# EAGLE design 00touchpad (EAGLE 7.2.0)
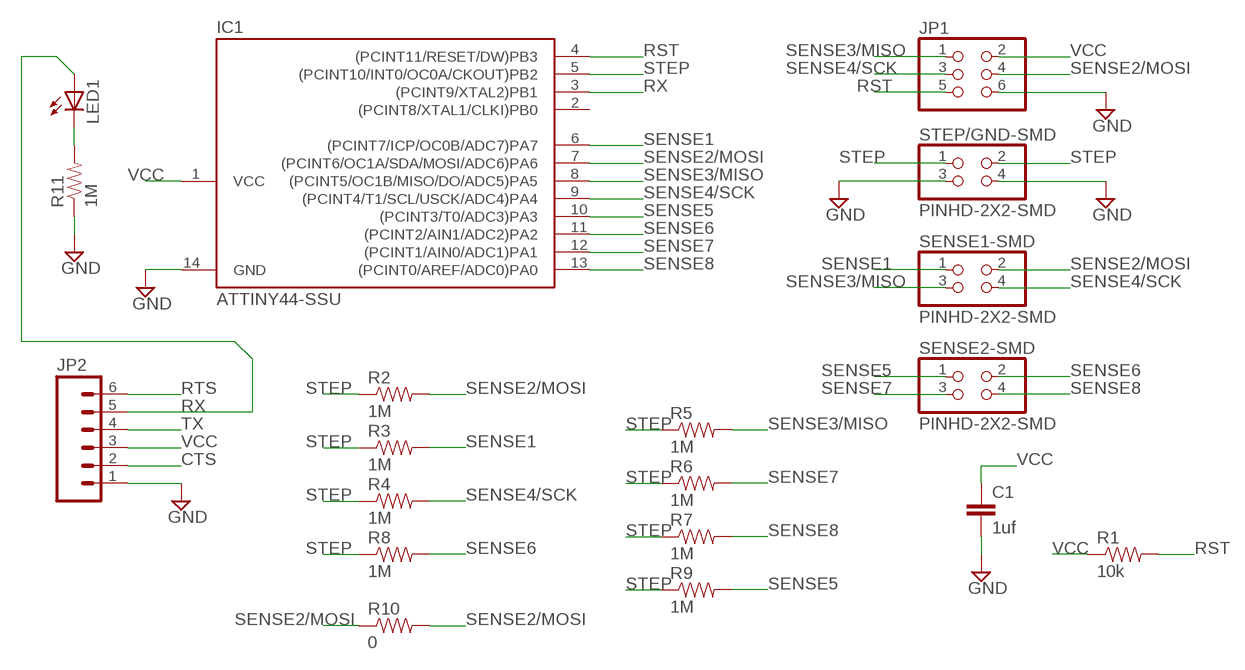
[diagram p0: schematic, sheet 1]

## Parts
C1  1uf  CAP1206  [1206]
IC1  ATTINY44-SSU  [SOIC14]
JP1  PINHD-2X3-SMD  [2X03SMD]
JP2  M06SMD  [1X06-SMD]
LED1  LEDSMT1206  [1206]
R1  10k  RESISTOR1206  [1206]
R2  1M  RESISTOR1206  [1206]
R3  1M  RESISTOR1206  [1206]
R4  1M  RESISTOR1206  [1206]
R5  1M  RESISTOR1206  [1206]
R6  1M  RESISTOR1206  [1206]
R7  1M  RESISTOR1206  [1206]
R8  1M  RESISTOR1206  [1206]
R9  1M  RESISTOR1206  [1206]
R10  0  RESISTOR1206  [1206]
R11  1M  RESISTOR1206  [1206]
SENSE1-SMD  PINHD-2X2-SMD  [2X02SMD]
SENSE2-SMD  PINHD-2X2-SMD  [2X02SMD]
STEP/GND-SMD  PINHD-2X2-SMD  [2X02SMD]

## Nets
CTS: JP2.2
GND: C1.2 IC1.14(GND) JP1.6 JP2.1 R11.1 STEP/GND-SMD.3 STEP/GND-SMD.4
N$3: LED1.C R11.2
RST: IC1.4((PCINT11/RESET/DW)PB3) JP1.5 R1.2
RTS: JP2.6
RX: IC1.3((PCINT9/XTAL2)PB1) JP2.5 LED1.A
SENSE1: IC1.6((PCINT7/ICP/OC0B/ADC7)PA7) R3.2 SENSE1-SMD.1
SENSE2/MOSI: IC1.7((PCINT6/OC1A/SDA/MOSI/ADC6)PA6) JP1.4 R2.2 R10.1 R10.2 SENSE1-SMD.2
SENSE3/MISO: IC1.8((PCINT5/OC1B/MISO/DO/ADC5)PA5) JP1.1 R5.2 SENSE1-SMD.3
SENSE4/SCK: IC1.9((PCINT4/T1/SCL/USCK/ADC4)PA4) JP1.3 R4.2 SENSE1-SMD.4
SENSE5: IC1.10((PCINT3/T0/ADC3)PA3) R9.2 SENSE2-SMD.1
SENSE6: IC1.11((PCINT2/AIN1/ADC2)PA2) R8.2 SENSE2-SMD.2
SENSE7: IC1.12((PCINT1/AIN0/ADC1)PA1) R6.2 SENSE2-SMD.3
SENSE8: IC1.13((PCINT0/AREF/ADC0)PA0) R7.2 SENSE2-SMD.4
STEP: IC1.5((PCINT10/INT0/OC0A/CKOUT)PB2) R2.1 R3.1 R4.1 R5.1 R6.1 R7.1 R8.1 R9.1 STEP/GND-SMD.1 STEP/GND-SMD.2
TX: JP2.4
VCC: C1.1 IC1.1(VCC) JP1.2 JP2.3 R1.1
Unconnected: IC1.2((PCINT8/XTAL1/CLKI)PB0)

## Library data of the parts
C1 = SparkFun:CAP: Capacitor
IC1 = fab:ATTINY44
JP1 = fab:PINHD-2X3-SMD: PIN HEADER
JP2 = SparkFun:M06: Header 6 Standard 6-pin 0.1" header. Use with straight break away headers (SKU : PRT-00116), right angle break away headers (PRT-00553), swiss pins (PRT-00743), machine pins (PRT-00117), and female headers (PRT-00115). Molex polarized connector foot print use with SKU : PRT-08094 with associated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
LED1 = 01_adafruit:LED: LED
R1-R11 = SparkFun:RESISTOR: Resistor
SENSE1-SMD SENSE2-SMD STEP/GND-SMD = fab:PINHD-2X2-SMD

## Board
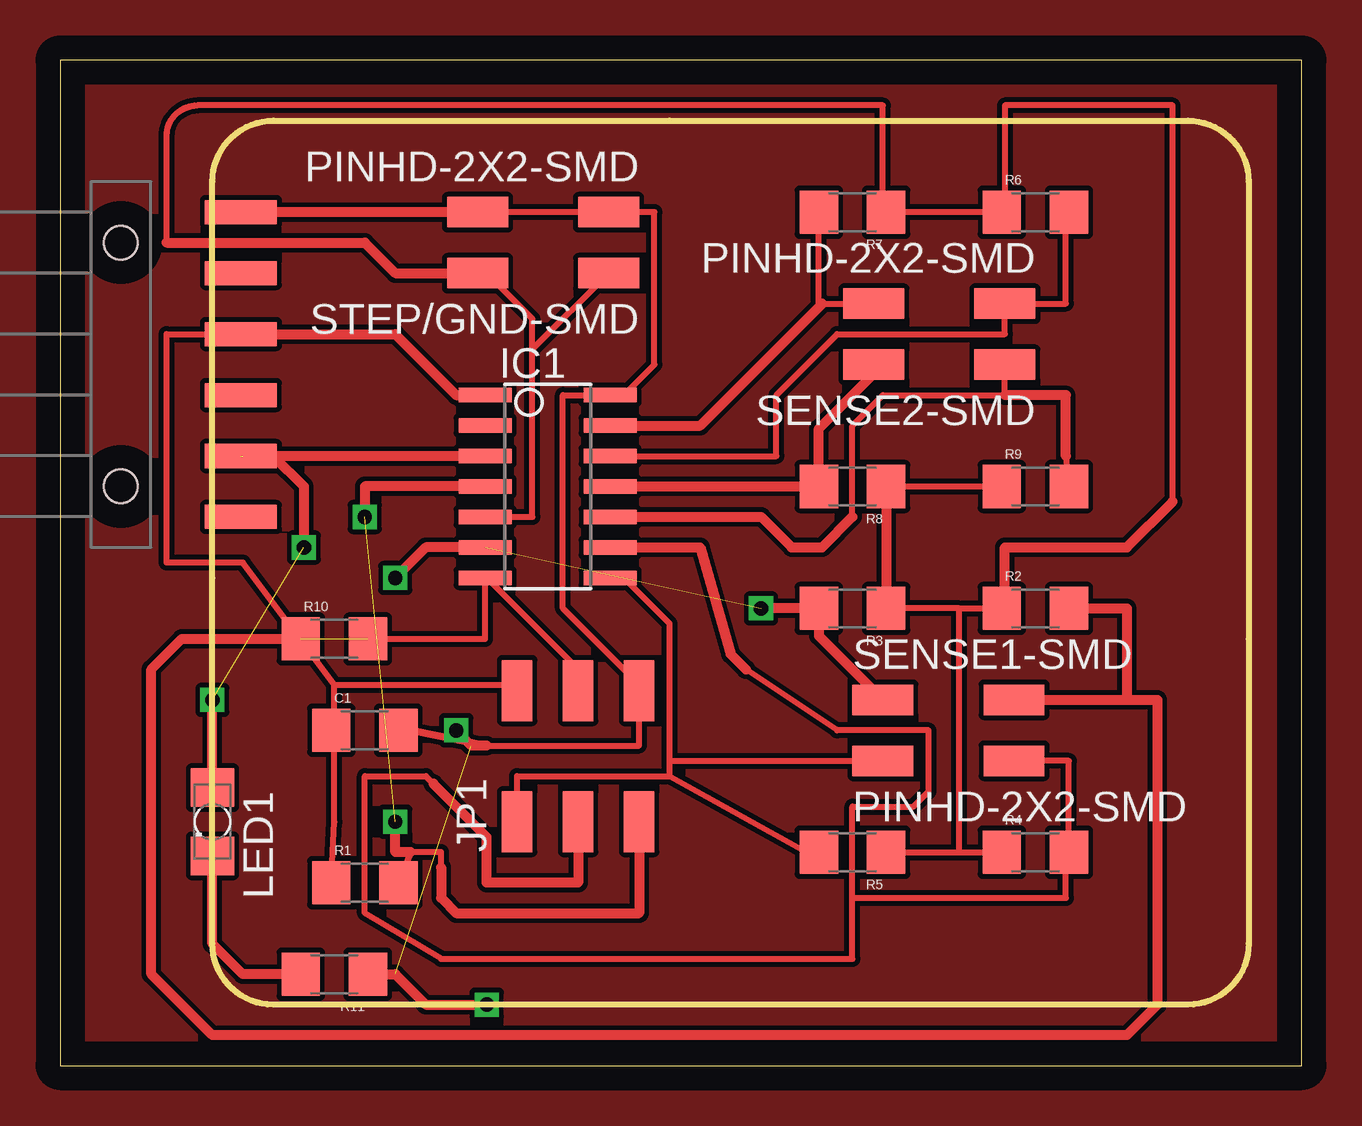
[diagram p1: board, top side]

Size 51.74 x 41.9 mm. Coordinates in mm from the lower left corner, seen from the top.
Outline: 0,0 51.74,0 51.74,41.9 0,41.9 0,0
Copper layers (1*16): Top 0.035mm / dielectric 1.5mm / Bottom 0.035mm
Design rules "default": minimum track width 10mil, minimum drill 24mil, track to track 8mil, track to pad 8mil, pad to pad 8mil, via to via 8mil, smd to smd 8mil, copper to edge 40mil, drill to drill 8mil, minimum pad ring 10mil, minimum via ring 8mil, stop-mask expansion 4mil, vias tented up to drill 0mil, thermal gap 10mil
Milling: area 6.3,2.5 to 49.5,39.4

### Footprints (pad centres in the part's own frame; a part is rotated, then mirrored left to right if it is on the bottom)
1206 = smd 1.6 x 1.8: 1 -1.4,0; 2 1.4,0
SOIC14 = smd 0.61 x 2.21: 1 -3.81,-2.603; 2 -2.54,-2.603; 3 -1.27,-2.603; 4 0,-2.603; 5 1.27,-2.603; 6 2.54,-2.603; 7 3.81,-2.603; 8 3.81,2.603; 9 2.54,2.603; 10 1.27,2.603; 11 0,2.603; 12 -1.27,2.603; 13 -2.54,2.603; 14 -3.81,2.603
2X03SMD = smd 2.54 x 1.27: 1 -2.54,2.54; 2 2.92,2.54; 3 -2.54,0; 4 2.92,0; 5 -2.54,-2.54; 6 2.92,-2.54
1X06-SMD = smd 1 x 3: 1 -6.35,5; 2 -3.81,5; 3 -1.27,5; 4 1.27,5; 5 3.81,5; 6 6.35,5 | hole 1.4: -5.08,0; 5.08,0
1206' = smd 1.6 x 1.803: A -1.422,0; C 1.422,0
2X02SMD = smd 2.54 x 1.27: 1 -2.54,1.27; 2 2.92,1.27; 3 -2.54,-1.27; 4 2.92,-1.27

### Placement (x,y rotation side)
C1  12.7,13.97 0 top
IC1  20.32,24.13 270 top
JP1  21.59,12.7 90 top
JP2  2.54,29.21 270 top
LED1  [1206']  6.35,10.16 270 top
R1  12.7,7.62 0 top
R2  40.64,19.05 0 top
R3  33.02,19.05 180 top
R4  40.64,8.89 0 top
R5  33.02,8.89 180 top
R6  40.64,35.56 0 top
R7  33.02,35.56 180 top
R8  33.02,24.13 180 top
R9  40.64,24.13 0 top
R10  11.43,17.78 0 top
R11  11.43,3.81 180 top
SENSE1-SMD  36.83,13.97 0 top
SENSE2-SMD  36.83,30.48 180 top
STEP/GND-SMD  20.32,34.29 180 top

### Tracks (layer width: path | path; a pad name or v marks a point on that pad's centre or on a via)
GND  (via drill 0.6)  (1 unrouted)
  Top 0.254: STEP/GND-SMD.4 STEP/GND-SMD.3 24.77,35.56 24.77,29.21 23.49,27.94 IC1.14 20.95,27.94 20.95,19.05 24.13,15.88 JP1.6 24.13,13.34 17.78,13.34 | C1.2 14.61,13.97
  Top 0.305: 14.61,13.97 17.78,13.34
  Top 0.406: R11.1 13.97,3.81 15.24,2.54 v17.78,2.54 | 17.78,13.34 17.14,13.34 v16.51,13.97 | STEP/GND-SMD.4 JP2.1
N$3
  Top 0.406: R11.2 7.62,3.81 6.35,5.08 LED1.C
N$4  (via drill 0.6)
  other vias: 6.35,15.24
N$5
  pour Top: -6.35,45.72 -6.35,-5.08 60.96,-5.08 60.96,48.26
RST  (via drill 0.6)  (1 unrouted)
  Top 0.254: 15.88,8.26 15.88,8.89 14.61,8.89 R1.2
  Top 0.406: IC1.4 12.7,24.13 v12.7,22.86 | 14.61,8.89 13.97,8.89 v13.97,10.16 | JP1.5 24.13,6.35 16.51,6.35 15.88,6.99 15.88,8.26
RX  (via drill 0.6)  (2 unrouted)
  Top 0.406: 7.62,25.4 8.89,25.4 10.16,24.13 v10.16,21.59 | LED1.A 6.35,15.24 | IC1.3 JP2.5
SENSE1  (via drill 0.6)  (1 unrouted)
  Top 0.254: R3.2 31.75,19.05
  Top 0.406: IC1.6 15.24,21.59 v13.97,20.32 | v29.21,19.05 R3.2 31.62,17.91 SENSE1-SMD.1
SENSE2/MOSI  (1 unrouted)
  Top 0.254: JP1.4 21.59,16.51 17.78,20.32 IC1.7 17.72,17.78 R10.2
  Top 0.406: SENSE1-SMD.2 44.45,15.24 | 44.45,15.24 45.72,15.24 45.72,2.54 44.45,1.27 6.35,1.27 3.81,3.81 3.81,16.51 5.08,17.78 R10.1 | R2.2 44.45,19.05 44.45,15.24
SENSE3/MISO
  Top 0.254: 25.4,12.06 31.11,8.89 R5.2 | 25.4,12.06 19.05,12.06 JP1.1 | 25.4,12.06 25.4,12.7 | 25.4,12.7 25.4,18.41 23.49,20.32 IC1.8 | 25.4,12.7 SENSE1-SMD.3
SENSE4/SCK
  Top 0.254: 28.57,16.51 32.38,13.97 36.2,13.97 36.2,11.43 35.56,10.79 33.02,10.79 33.02,6.99 | 17.14,10.16 15.56,11.75 15.24,12.06 12.7,12.06 12.7,6.35 15.88,4.45 33.02,4.45 33.02,6.99 | SENSE1-SMD.4 42.04,12.7 R4.2 41.91,8.89 41.91,6.99 33.02,6.99
  Top 0.406: IC1.9 26.67,21.59 27.94,17.14 28.57,16.51 | JP1.3 21.59,7.62 17.78,7.62 17.78,9.53 15.56,11.75
SENSE5
  Top 0.254: SENSE2-SMD.1 39.37,27.94 34.29,27.94 33.02,26.67 33.02,22.86 | 41.91,25.4 R9.2
  Top 0.406: IC1.10 29.21,22.86 30.48,21.59 31.75,21.59 33.02,22.86 | 41.91,25.4 41.91,27.94 39.37,27.94
SENSE6
  Top 0.406: IC1.11 R8.2 31.62,26.54 34.29,29.21 SENSE2-SMD.2
SENSE7
  Top 0.254: R6.2 41.91,35.56 41.91,31.75 SENSE2-SMD.3 39.37,30.48 32.38,30.48 29.84,27.94 29.84,25.4 IC1.12
SENSE8
  Top 0.254: R7.2 31.62,31.75 31.75,31.75 SENSE2-SMD.4
  Top 0.406: IC1.13 26.67,26.67 31.75,31.75
STEP
  Top 0.254: 19.68,29.84 19.68,31.11 17.78,33.02 STEP/GND-SMD.2 | 19.68,29.84 19.68,22.86 IC1.5 | 19.68,29.84 STEP/GND-SMD.1 | R8.1 R9.1 | R5.1 37.46,8.89 | 37.46,8.89 R4.1 | 37.46,19.05 R3.1 34.29,19.05 | 37.46,19.05 R2.1 39.37,19.05 | 37.46,8.89 37.46,19.05 | 46.35,23.5 46.35,40.01 39.37,40.01 39.37,35.56 R6.1 R7.1 34.29,35.56 34.29,40.01 5.71,40.01 arc90 4.45,38.73 4.45,34.29
  Top 0.406: 39.37,19.05 39.37,21.59 44.45,21.59 46.35,23.5 | R8.1 R3.1 | 4.45,34.29 12.7,34.29 13.97,33.02 STEP/GND-SMD.2
VCC
  Top 0.254: 11.43,13.97 11.43,10.16 R1.1 | 11.43,15.88 19.05,15.88 JP1.2 | 11.43,13.97 C1.1 | 11.43,13.97 11.43,15.88 | 11.43,15.88 7.62,20.95 4.45,20.95 4.45,30.48 JP2.3
  Top 0.406: JP2.3 13.97,30.48 16.51,27.94 IC1.1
